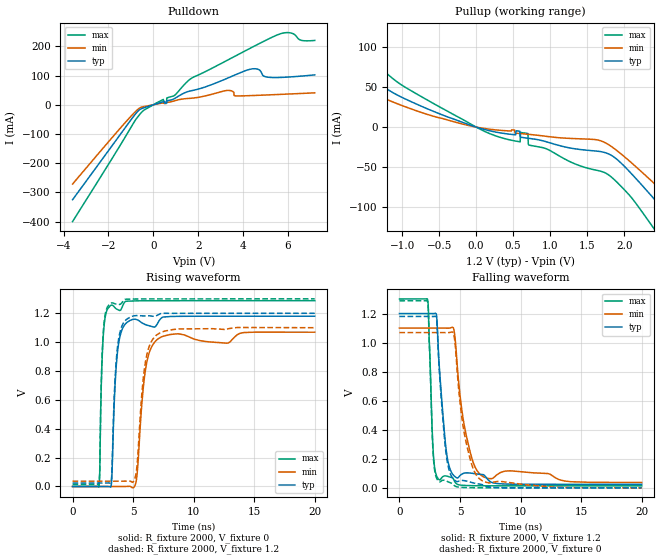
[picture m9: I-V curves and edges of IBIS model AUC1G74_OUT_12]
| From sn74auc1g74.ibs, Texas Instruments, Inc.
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[Model]   AUC1G74_OUT_12
Model_type  Output
Vref =   0
Rref =   2000
Cref =   15p
Vmeas =   0.6
| variable   typ   min   max
C_comp   4.63pF   0.44pF   7.09pF
| C_pullup   3.96pF   0.44pF   7.09pF
| C_pulldown   5.30pF   1.35pF   6.29pF
[Temperature Range]   40   100   -40
| Ambient temperature   25   85   -40
[Voltage range]   1.2   1.1   1.3
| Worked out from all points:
|   slope of the pulldown table from 0 to 0.18 V, typ, clamps not added: 41.8 ohm
|   slope of the pullup table from 0 to 0.18 V, typ, clamps not added: 39 ohm
|   rising waveform, R_fixture 2000, V_fixture 0: 20-80 % time 418ps typ, 675ps min, 250ps max; typ from 0 V to 1.18 V
|   falling waveform, R_fixture 2000, V_fixture 1.2: 20-80 % time 658ps typ, 1.1ns min, 324ps max; typ from 1.2 V to 0.024 V
|   rising waveform, R_fixture 2000, V_fixture 1.2: 20-80 % time 404ps typ, 656ps min, 245ps max; typ from 0.024 V to 1.2 V
|   falling waveform, R_fixture 2000, V_fixture 0: 20-80 % time 646ps typ, 1.07ns min, 320ps max; typ from 1.18 V to 0 V
[Pulldown]
| AUC1G74_OUT_12
|   Voltage   I(typ)   I(min)   I(max)
-3.6V     -324.8mA   -271.2mA   -399.5mA
-860mV    -37.72mA   -28.15mA   -59.7mA
-430mV    -10.35mA   -6.385mA   -19.13mA
590mV     6.038mA    8.092mA    8.62mA
605mV     6.519mA    8.238mA    23.43mA
1.675V    47.71mA    22.31mA    89.32mA
3.275V    89.89mA    48.93mA    151.3mA
4.32V     121.7mA    31.34mA    193.3mA
5.53V     93.22mA    35.11mA    239.1mA
6.085V    95.19mA    36.97mA    246.4mA
6.58V     98.02mA    38.67mA    220.8mA
7.2V      102.2mA    40.86mA    220mA
[Pullup]
| AUC1G74_OUT_12
|   Voltage   I(typ)   I(min)   I(max)
-3.6V     246.3mA    203.7mA    293.5mA
-2.66V    159.1mA    124.9mA    201.9mA
-1.9V     95.07mA    70.9mA     129mA
-1.04V    38.96mA    28.34mA    54.82mA
10mV      -294.5uA   -174.9uA   -513.2uA
700mV     -14.01mA   -9.053mA   -8.046mA
715mV     -14.2mA    -9.18mA    -22.56mA
1.785V    -33.51mA   -21.79mA   -59.64mA
2.375V    -86.88mA   -67.97mA   -123.6mA
2.62V     -112.8mA   -89.28mA   -155.6mA
3.25V     -180.4mA   -145.6mA   -236.9mA
7.2V      -602.3mA   -508.1mA   -734.3mA
[Ramp]
| AUC1G74_OUT_12
| variable   typ   min   max
dV/dt_r   0.71/4.20E-10   0.65/6.81E-10   0.78/2.51E-10
dV/dt_f   0.71/6.61E-10   0.64/1.10E-09   0.77/3.25E-10
R_load = 2000
[Rising Waveform]
| AUC1G74_OUT_12
R_fixture =   2000
C_fixture =   0
L_fixture =   0
V_fixture =   0
V_fixture_min = 0
V_fixture_max = 0
|   Time   V(typ)   V(min)   V(max)
0s        7.653nV    32.85nV    737.2pV
2.175ns   -167.5nV   80.75nV    -4.501mV
2.525ns   -7.111uV   -369.2nV   1.03V
3.115ns   -2.678mV   162.1nV    1.252V
3.69ns    915mV      -5.926uV   1.227V
4.49ns    1.137V     516.4uV    1.284V
5.255ns   1.157V     35.32mV    1.286V
6.01ns    1.122V     802.6mV    1.287V
7ns       1.127V     1.019V     1.287V
20ns      1.18V      1.069V     1.287V
[Falling Waveform]
| AUC1G74_OUT_12
R_fixture =   2000
C_fixture =   0
L_fixture =   0
V_fixture =   1.2
V_fixture_min = 1.1
V_fixture_max = 1.3
|   Time   V(typ)   V(min)   V(max)
0s        1.2V       1.1V       1.3V
2.32ns    1.2V       1.1V       1.296V
2.795ns   1.2V       1.1V       240.5mV
3.055ns   1.196V     1.1V       84.87mV
3.255ns   884.9mV    1.1V       57.96mV
4.18ns    128.3mV    1.101V     73.93mV
4.54ns    80.48mV    1.067V     46.37mV
5.49ns    103.2mV    372.5mV    16.29mV
6.765ns   92.22mV    85.55mV    14.36mV
20ns      24.06mV    36.81mV    13.89mV
[Rising Waveform]
| AUC1G74_OUT_12
R_fixture =   2000
C_fixture =   0
L_fixture =   0
V_fixture =   1.2
V_fixture_min = 1.1
V_fixture_max = 1.3
|   Time   V(typ)   V(min)   V(max)
0s        23.98mV    36.62mV    13.86mV
2.175ns   23.98mV    36.62mV    9.447mV
2.52ns    23.97mV    36.62mV    1.045V
3.115ns   22.84mV    36.62mV    1.267V
3.68ns    941.2mV    36.62mV    1.264V
4.46ns    1.158V     37mV       1.298V
5.225ns   1.184V     82.62mV    1.299V
5.98ns    1.182V     842.3mV    1.3V
6.94ns    1.184V     1.05V      1.3V
20ns      1.2V       1.1V       1.3V
[Falling Waveform]
| AUC1G74_OUT_12
R_fixture =   2000
C_fixture =   0
L_fixture =   0
V_fixture =   0
V_fixture_min = 0
V_fixture_max = 0
|   Time   V(typ)   V(min)   V(max)
0s        1.18V      1.069V     1.287V
2.315ns   1.18V      1.069V     1.285V
2.79ns    1.179V     1.069V     226.1mV
3.055ns   1.175V     1.069V     69.36mV
3.24ns    880.3mV    1.069V     44.64mV
4.15ns    108.7mV    1.069V     36.82mV
4.53ns    55mV       1.037V     15.83mV
5.445ns   48.37mV    337.2mV    2.051mV
6.685ns   24.94mV    57.01mV    470uV
20ns      73.17uV    89.98uV    26.74uV
